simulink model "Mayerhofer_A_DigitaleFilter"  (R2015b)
settings: Solver=VariableStepAuto  StartTime=0.0  StopTime=1  RelTol=1e-3
libraries: dsparch4 x1, dspsrcs4 x1

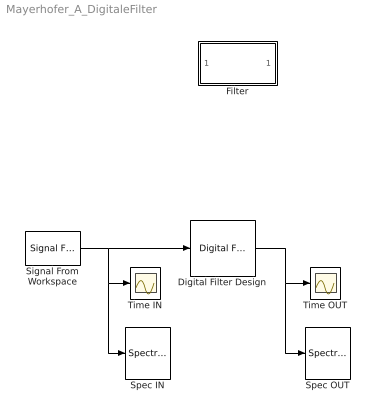
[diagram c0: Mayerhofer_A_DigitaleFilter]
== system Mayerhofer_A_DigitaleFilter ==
  Digital Filter Design : dsparch4/Digital Filter Design  mwdsp_browser_bugfix_var=off
  Filter : Subsystem  Tag=FilterWizardSubSystem
  Signal From Workspace : dspsrcs4/Signal From Workspace  X=signal7  Ts=1/8000  nsamps=1  OutputAfterFinalValue=Cyclic repetition  ignoreOrWarnInputAndFrameLengths=on  OutputFrames=off
  Spec IN : SpectrumAnalyzer
  Spec OUT : SpectrumAnalyzer
  Time IN : Scope
  Time OUT : Scope
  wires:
  Signal From Workspace/1 -> Spec IN/1, Time IN/1, Digital Filter Design/1
  Digital Filter Design/1 -> Spec OUT/1, Time OUT/1

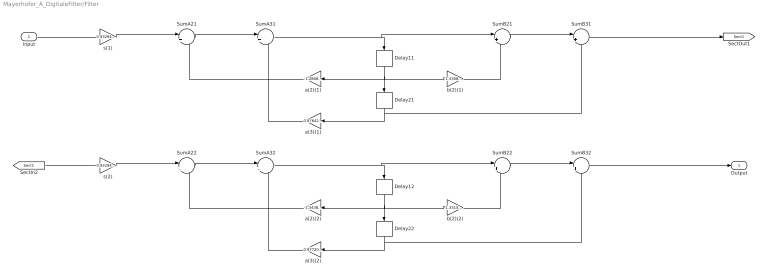
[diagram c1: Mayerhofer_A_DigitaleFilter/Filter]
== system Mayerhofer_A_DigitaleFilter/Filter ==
  Input : Inport
  Delay{11..12,21..22} (4 alike) : Delay  DelayLength=1  InitialCondition=0
  SumA{21..22,31..32} (4 alike) : Sum  Inputs=|+-  RndMeth=Nearest
  SumB{21..22,31..32} (4 alike) : Sum  Inputs=|++  RndMeth=Nearest
  a(2)(1) : Gain  Gain=-1.2868250974445234  ParamDataTypeStr=double  RndMeth=Nearest
  a(2)(2) : Gain  Gain=-1.3438056825526017  ParamDataTypeStr=double  RndMeth=Nearest
  a(3)(1) : Gain  Gain=0.97642787295864619  ParamDataTypeStr=double  RndMeth=Nearest
  a(3)(2) : Gain  Gain=0.97720971489810515  ParamDataTypeStr=double  RndMeth=Nearest
  b(2)(1) : Gain  Gain=-1.3308661944188238  ParamDataTypeStr=double  RndMeth=Nearest
  b(2)(2) : Gain  Gain=-1.3315758737107264  ParamDataTypeStr=double  RndMeth=Nearest
  s(1) : Gain  Gain=0.93294784952258414  ParamDataTypeStr=double  RndMeth=Nearest
  s(2) : Gain  Gain=0.93294784952258414  ParamDataTypeStr=double  RndMeth=Nearest
  Output : Outport
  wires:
  Input/1 -> s(1)/1
  s(1)/1 -> SumA21/1
  SumA21/1 -> SumA31/1
  SumA31/1 -> SumB21/1, Delay11/1
  SumB21/1 -> SumB31/1
  SumB31/1 -> [Sect1]
  a(2)(1)/1 -> SumA21/2
  Delay11/1 -> a(2)(1)/1, b(2)(1)/1, Delay21/1
  b(2)(1)/1 -> SumB21/2
  a(3)(1)/1 -> SumA31/2
  Delay21/1 -> a(3)(1)/1, SumB31/2
  [Sect1] -> s(2)/1
  s(2)/1 -> SumA22/1
  SumA22/1 -> SumA32/1
  SumA32/1 -> SumB22/1, Delay12/1
  SumB22/1 -> SumB32/1
  SumB32/1 -> Output/1
  a(2)(2)/1 -> SumA22/2
  Delay12/1 -> a(2)(2)/1, b(2)(2)/1, Delay22/1
  b(2)(2)/1 -> SumB22/2
  a(3)(2)/1 -> SumA32/2
  Delay22/1 -> a(3)(2)/1, SumB32/2
